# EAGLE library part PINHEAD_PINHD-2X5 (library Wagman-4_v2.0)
PIN HEADER
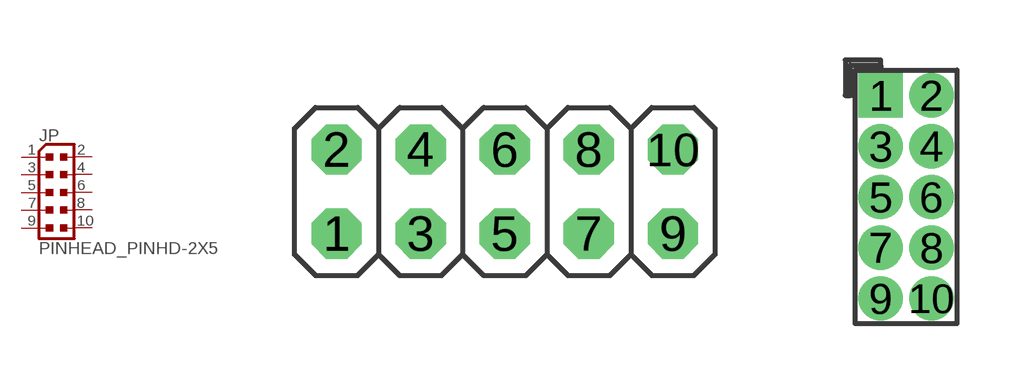
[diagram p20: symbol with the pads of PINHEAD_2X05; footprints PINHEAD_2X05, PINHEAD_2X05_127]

Designator prefix JP

## PINHEAD_PINHD-2X5  [PINHEAD_2X05]
1  1  pas
2  2  pas
3  3  pas
4  4  pas
5  5  pas
6  6  pas
7  7  pas
8  8  pas
9  9  pas
10  10  pas

## PINHEAD_PINHD-2X5PASSO127  [PINHEAD_2X05_127]
Pads as for PINHEAD_2X05

## Footprint PINHEAD_2X05 (pad centres in mm)
PIN HEADER
drill 1.016 octagon: 1 -5.08,-1.27; 2 -5.08,1.27; 3 -2.54,-1.27; 4 -2.54,1.27; 5 0,-1.27; 6 0,1.27; 7 2.54,-1.27; 8 2.54,1.27; 9 5.08,-1.27; 10 5.08,1.27

## Footprint PINHEAD_2X05_127 (pad centres in mm)
drill 0.6 pad 1.016 square: 1 -0.635,2.54
drill 0.6 pad 1.016: 2 0.635,2.54; 3 -0.635,1.27; 4 0.635,1.27; 5 -0.635,0; 6 0.635,0; 7 -0.635,-1.27; 8 0.635,-1.27; 9 -0.635,-2.54; 10 0.635,-2.54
